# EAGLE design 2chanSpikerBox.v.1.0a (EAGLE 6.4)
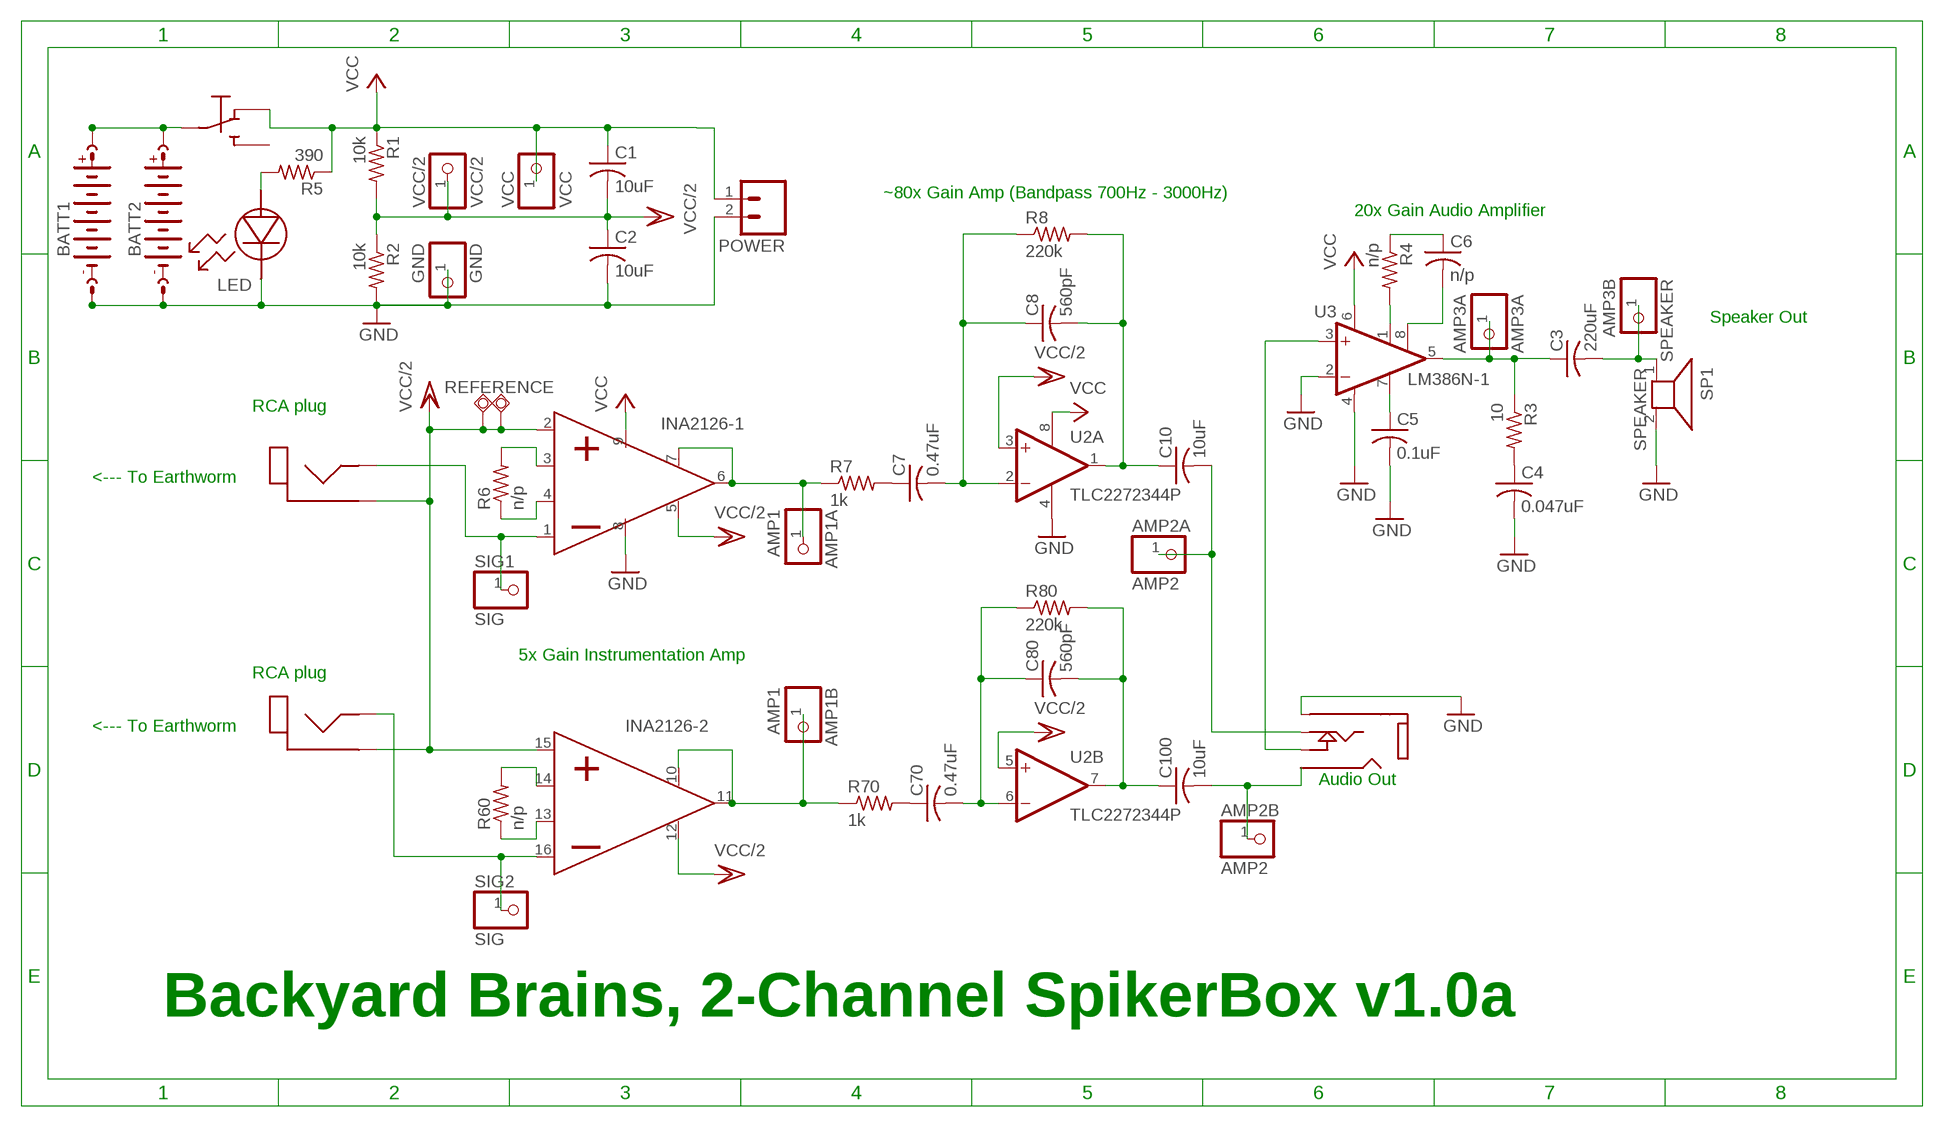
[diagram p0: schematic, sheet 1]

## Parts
AMP1A  AMP1  PINHD-1X1  [1X01]
AMP1B  AMP1  PINHD-1X1  [1X01]
AMP2A  AMP2  PINHD-1X1  [1X01]
AMP2B  AMP2  PINHD-1X1  [1X01]
AMP3A  AMP3A  PINHD-1X1  [1X01]
BATT1  9V-BATT-HOLDERSTANDS  [KEYSTONE-593-594]
BATT2  9V-BATT-HOLDERHEADERS  [1X02]
C1  10uF  C-US050-024X044  [C050-024X044]
C2  10uF  C-US050-024X044  [C050-024X044]
C3  220uF  C-US050-050X075  [C050-050X075]
C4  0.047uF  C-US050-024X044  [C050-024X044]
C5  0.1uF  C-US050-024X044  [C050-024X044]
C6  n/p  C-US050-030X075  [C050-030X075]
C7  0.47uF  C-US050-024X044  [C050-024X044]
C8  560pF  C-US050-024X044  [C050-024X044]
C10  10uF  C-US050-030X075  [C050-030X075]
C70  0.47uF  C-US050-024X044  [C050-024X044]
C80  560pF  C-US050-024X044  [C050-024X044]
C100  10uF  C-US050-030X075  [C050-030X075]
GND  GND  PINHD-1X1  [1X01]
J1  RCA  [RCJ]
J2  RCA  [RCJ]
J4  AUD  AUDIOJACK3.5MM  [AUDIO-JACK]
LED  LEDSSF-LXH104GD  [SSF-LXH104GD]
POWER  M02PTH  [1X02]
R1  10k  R-US_0411/3V  [0411V]
R2  10k  R-US_0411/3V  [0411V]
R3  10  R-US_0309/V  [0309V]
R4  n/p  R-US_0309/V  [0309V]
R5  390  R-US_0309/V  [0309V]
R6  n/p  R-US_0309/V  [0309V]
R7  1k  R-US_0309/V  [0309V]
R8  220k  R-US_0309/V  [0309V]
R60  n/p  R-US_0309/V  [0309V]
R70  1k  R-US_0309/V  [0309V]
R80  220k  R-US_0309/V  [0309V]
REFERENCE  TPSQTP20SQ  [TP20SQ]
REFERENCE1  TPSQTP20SQ  [TP20SQ]
SIG1  SIG  PINHD-1X1  [1X01]
SIG2  SIG  PINHD-1X1  [1X01]
SP1  SPEAKER  [1X02]
SPEAKER  AMP3B  PINHD-1X1  [1X01]
SW1  SWITCH  [SWITCH_THROUGHHOLE]
U1  INA2126  [DIL16]
U2  TLC2272344P  [DIL08]
U3  LM386N-1  [DIL08]
VCC  VCC  PINHD-1X1  [1X01]
VCC/2  VCC/2  PINHD-1X1  [1X01]

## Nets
GND: BATT1.GND$1(-) BATT2.2(-) C2.2 C4.2 C5.2 GND.1 J4.1(SHIELD) LED.CATHODE POWER.2 R2.2 SP1.2 U1.8(PGND) U2.4(A:V-) U3.2(-IN) U3.4(GND)
N$1: AMP2B.1 C100.2 J4.3(INPUTB)
N$2: AMP3A.1 C3.1 R3.1 U3.5(OUT)
N$3: AMP1B.1 R70.1 U1.10(PSENSE) U1.11(POUT)
N$5: C7.1 R7.2
N$6: C4.1 R3.2
N$7: AMP2A.1 C10.2 J4.2(INPUTA)
N$8: C5.1 U3.7(BYPASS)
N$9: C7.2 C8.1 R8.1 U2.2(A:-IN)
N$10: C6.1 R4.1
N$11: R4.2 U3.1(GAIN)
N$12: C6.2 U3.8(GAIN)
N$13: R6.2 U1.3(PG1)
N$14: LED.ANODE R5.2
N$15: J2.SIG SIG2.1 U1.16(P-)
N$16: R6.1 U1.4(PG2)
N$17: AMP1A.1 R7.1 U1.6(POUT) U1.7(PSENSE)
N$18: R60.2 U1.14(PG1)
N$19: C70.1 R70.2
N$20: C70.2 C80.1 R80.1 U2.6(B:-IN)
N$21: J1.SIG SIG1.1 U1.1(P-)
N$22: R60.1 U1.13(PG2)
N$23: C8.2 C10.1 R8.2 U2.1(A:OUT)
N$24: C3.2 SP1.1 SPEAKER.1
N$28: J4.4(SPEAKEROUT) U3.3(+IN)
N$29: C80.2 C100.1 R80.2 U2.7(B:OUT)
V9HOT: BATT1.+9V$1(+) BATT2.1(+) SW1.P2
VCC: C1.1 POWER.1 R1.1 R5.1 SW1.P3 U1.9(PVCC) U2.8(A:V+) U3.6(VS) VCC.1
VCC/2: C1.2 C2.1 J1.GND$1(GND) J2.GND$1(GND) R1.2 R2.1 REFERENCE1.TP REFERENCE.TP U1.2(P+) U1.5(PREF) U1.12(PREF) U1.15(P+) U2.3(A:+IN) U2.5(B:+IN) VCC/2.1
Unconnected: SW1.P1

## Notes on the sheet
- ~80x Gain Amp (Bandpass 700Hz - 3000Hz)
- 20x Gain Audio Amplifier
- Speaker Out
- RCA plug
- INA2126-1
- <--- To Earthworm
- 5x Gain Instrumentation Amp
- RCA plug
- <--- To Earthworm | INA2126-2
- Audio Out
- Backyard Brains, 2-Channel SpikerBox v1.0a

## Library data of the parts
AMP1A AMP1B AMP2A AMP2B AMP3A GND SIG1 SIG2 SPEAKER VCC VCC/2 = pinhead:PINHD-1X1: PIN HEADER
BATT1 = byb:9V-BATT-HOLDER; DIGIKEY: 593K-ND, 594K-ND; MANUFACTURER: KEYSTONE ELECTRONICS; PARTNO: 593,594
BATT2 = byb:9V-BATT-HOLDER; DIGIKEY: N145-ND; MANUFACTURER: ENERGIZER BATTERY COMPANY; PARTNO: EN22
C1 C2 = resistor:C-US: CAPACITOR, American symbol; DIGIKEY: P986-ND; MANUFACTURER: Panasonic - ECG; PARTNO: ECE-A1HKSR22
C3 = resistor:C-US: CAPACITOR, American symbol; DIGIKEY: 565-1674-ND; MANUFACTURER: UNITED CHEMI-CON; PARTNO: EKZE250ELL221MHB5D
C4 = resistor:C-US: CAPACITOR, American symbol; DIGIKEY: BC1099CT-ND; MANUFACTURER: VISHAY/BC COMPONENTS; PARTNO: K473K15X7RF5TH5
C5 = resistor:C-US: CAPACITOR, American symbol; DIGIKEY: BC1148CT-ND; MANUFACTURER: Vishay/BC Components; PARTNO: K104Z15Y5VE5TL2
C6 C10 C100 = resistor:C-US: CAPACITOR, American symbol; DIGIKEY: P966-ND; MANUFACTURER: Panasonic - ECG; PARTNO: ECE-A1CKS100
C7 C70 = resistor:C-US: CAPACITOR, American symbol; DIGIKEY: BC1150CT-ND; MANUFACTURER: Vishay/BC Components; PARTNO: K474Z20Y5VE5TL2
C8 C80 = resistor:C-US: CAPACITOR, American symbol; DIGIKEY: BC1022CT-ND; MANUFACTURER: Vishay/BC Components; PARTNO: K561J15C0GF5TL2
J1 J2 = byb:RCA: RCA Edge Connector; DIGIKEY: CP-1403-ND; MANUFACTURER: CUI Inc; PARTNO: RCJ-014
J4 = byb:AUDIOJACK: 1/8" Audio Jack; DIGIKEY: CP1-3524NG-ND; MANUFACTURER: CUI Inc; PARTNO: SJ1-3524NG
LED = byb:LED: SIDE LED (Green); DIGIKEY: 67-1037-ND; MANUFACTURER: LUMEX OPTO/COMPONENTS INC; PARTNO: SSF-LXH104GD
POWER = SparkFun:M02: Header 2
R1 R2 = resistor:R-US_: RESISTOR, American symbol; DIGIKEY: P10KBACT-ND; MANUFACTURER: Panasonic - ECG; PARTNO: ERD-S2TJ103V
R3 = resistor:R-US_: RESISTOR, American symbol; DIGIKEY: P10BACT-ND; MANUFACTURER: Panasonic - ECG; PARTNO: ERD-S2TJ100V
R4 = resistor:R-US_: RESISTOR, American symbol; DIGIKEY: CD14ZT0R00CT-ND; MANUFACTURER: Stackpole Electronics; PARTNO: CD14ZT0R00
R5 = resistor:R-US_: RESISTOR, American symbol; DIGIKEY: CF14JT390RCT-ND; MANUFACTURER: Stackpole Electronics; PARTNO: CF14JT390R
R6 R60 = resistor:R-US_: RESISTOR, American symbol; DIGIKEY: P68KBACT-ND; MANUFACTURER: Panasonic - ECG; PARTNO: ERD-S2TJ683V
R7 R70 = resistor:R-US_: RESISTOR, American symbol; DIGIKEY: P1.0KBACT-ND; MANUFACTURER: Panasonic - ECG; PARTNO: ERD-S2TJ102V
R8 R80 = resistor:R-US_: RESISTOR, American symbol; DIGIKEY: P220KCACT-ND; MANUFACTURER: Panasonic - ECG; PARTNO: ERO-S2PHF2203
REFERENCE REFERENCE1 = testpad:TPSQ: Test pad
SP1 = byb:SPEAKER: SPEAKER; DIGIKEY: 102-1554-ND; MANUFACTURER: CUI Inc; PARTNO: CLS0271M-L152
SW1 = byb:SWITCH: Toggle Switch
U1 = byb:INA2126
U2 = byb:TLC2272: Dual Operational Amplifier Low Power, Single-Supply, Rail-To-Rail Operational Amplifier Source: http://focus.ti.com/lit/ds/symlink/opa2345.pdf http://focus.ti.com .. opa241.pdf http://focus.ti.com/lit/ds/symlink/opa2134.pdf; DIGIKEY: 296-1812-5-ND; MANUFACTURER: TEXAS INSTRUMENTS; PARTNO: TLC2272CP
U3 = byb:LM386?-*: Low Voltage Audio Power Amplifier Source: http://cache.national.com/ds/LM/LM386.pdf; DIGIKEY: LM386N-3-ND; MANUFACTURER: NATIONAL SEMICONDUCTOR; PARTNO: LM386N-3/NOPB

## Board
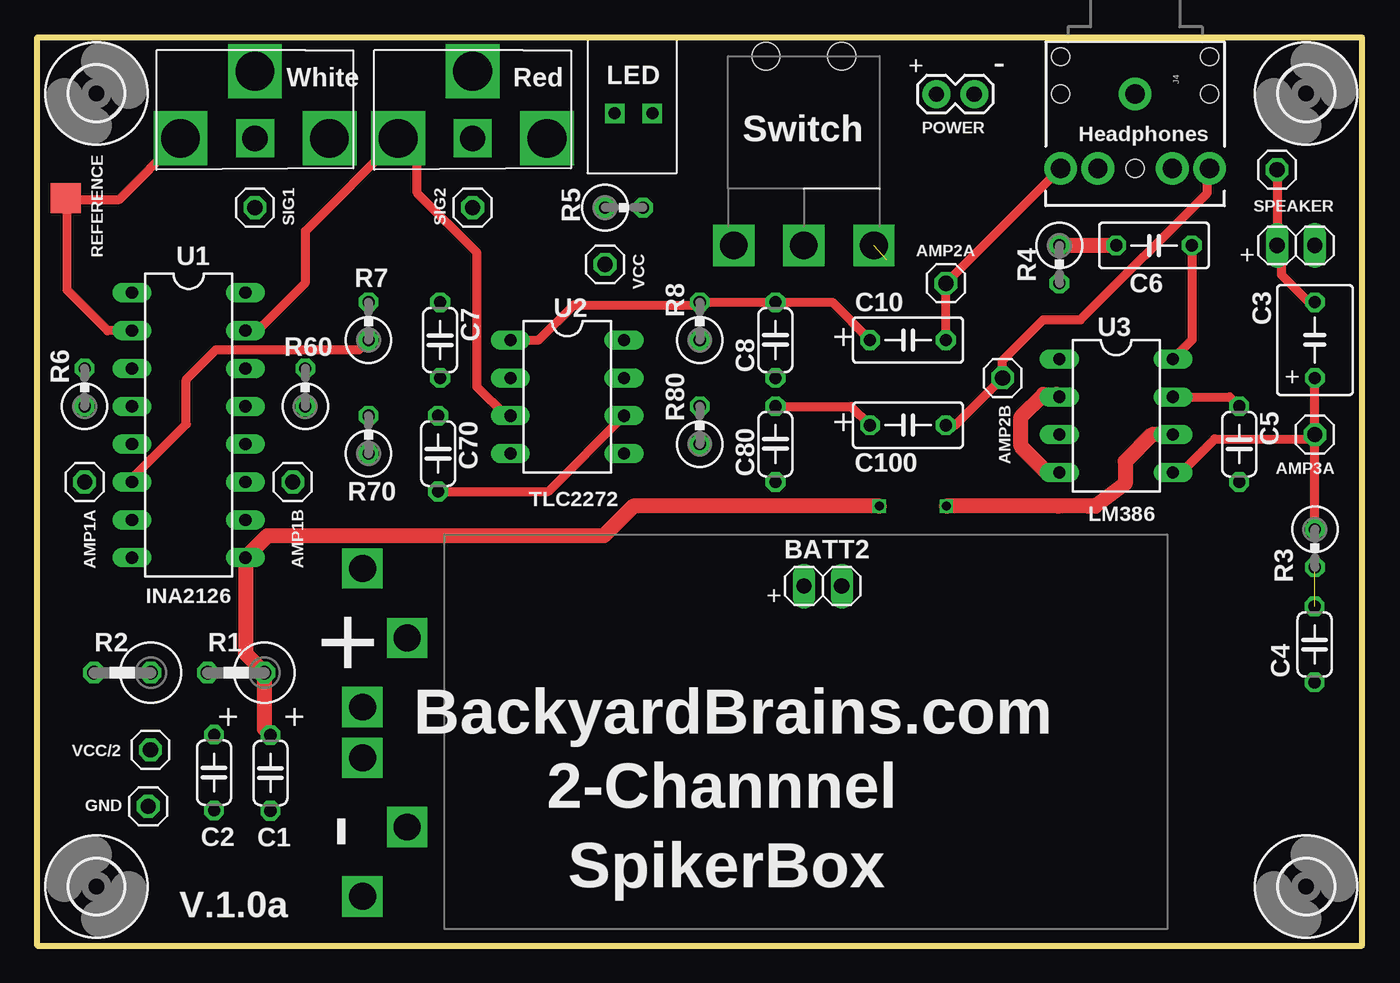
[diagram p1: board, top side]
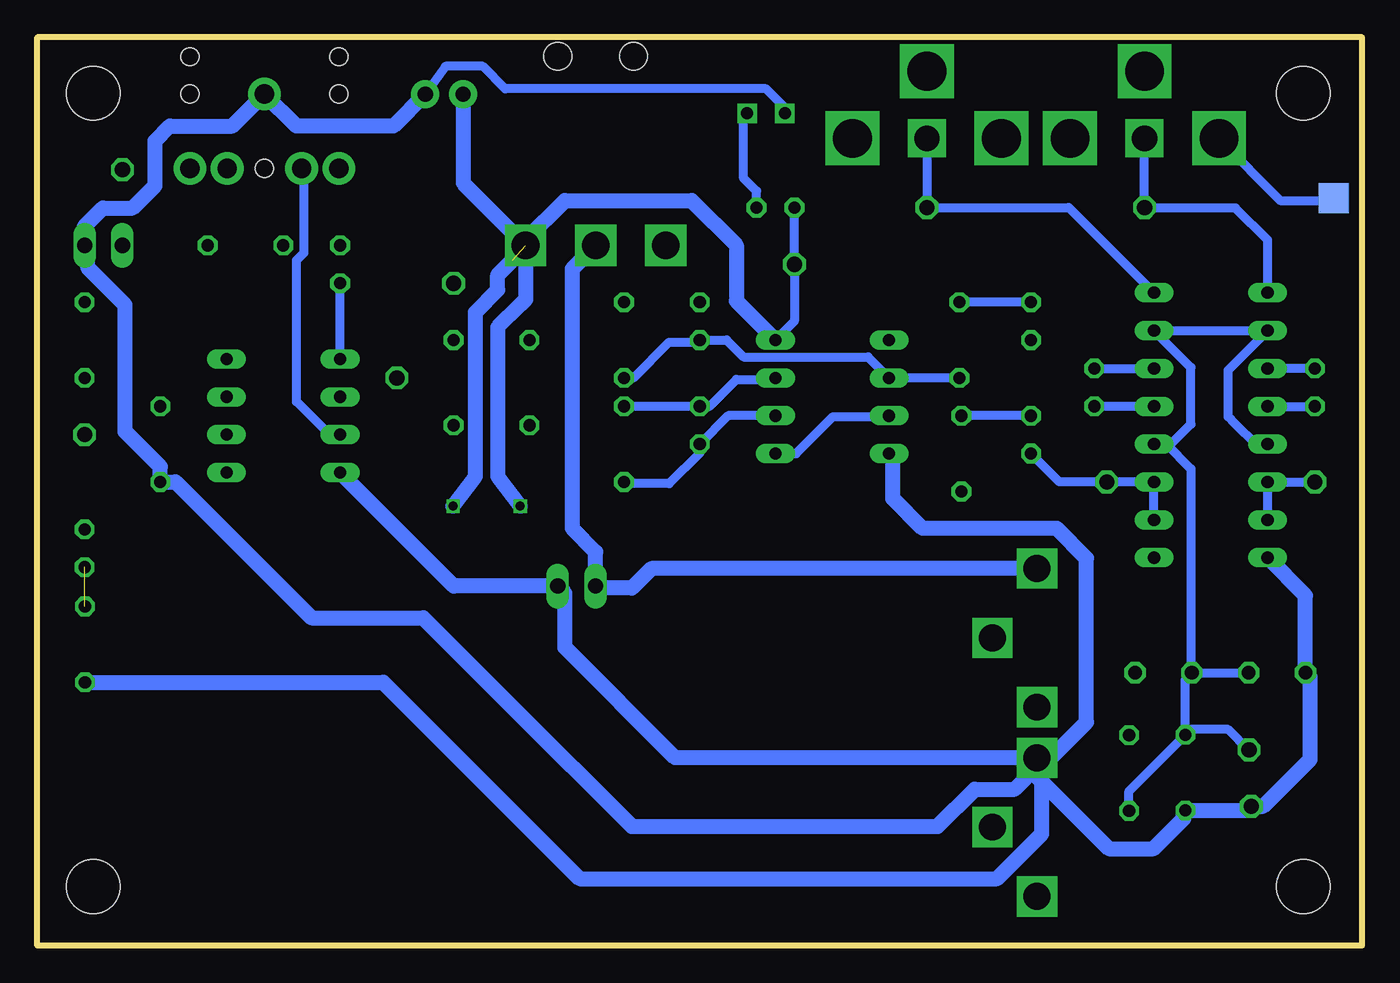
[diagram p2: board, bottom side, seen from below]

Size 88.9 x 60.96 mm. Coordinates in mm from the lower left corner, seen from the top.
Outline: 0,0 0,60.96 88.9,60.96 88.9,0 0,0
Copper layers (1*16): Top 0.035mm / dielectric 1.5mm / Bottom 0.035mm
Design rules "default": minimum track width 6mil, minimum drill 12mil, track to track 6mil, track to pad 6mil, pad to pad 6mil, via to via 6mil, smd to smd 0mil, copper to edge 10mil, drill to drill 10mil, minimum pad ring 10mil, minimum via ring 6mil, stop-mask expansion 2mil, vias tented up to drill 100mil, thermal gap 10mil

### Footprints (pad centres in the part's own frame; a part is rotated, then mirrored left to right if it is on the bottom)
1X01 = drill 1.016 octagon: 1 0,0
KEYSTONE-593-594 = drill 1.8 square: +9V$1 -10.7,1.5; +9V$2 -6.05,4.5; +9V$3 -1.4,1.5; GND$1 2,1.5; GND$2 6.65,4.5; GND$3 11.3,1.5
1X02 = drill 1.016 long: 1 -1.27,0; 2 1.27,0
C050-024X044 = drill 0.813 octagon: 1 -2.54,0; 2 2.54,0
C050-050X075 = drill 0.813 octagon: 1 -2.54,0; 2 2.54,0
C050-030X075 = drill 0.813 octagon: 1 -2.54,0; 2 2.54,0
3,6 = hole 3.6: 0,0
RCJ = drill 2.6 square: GND$1 -5,-4.5; GND$2 0,0; GND$3 5,-4.5 | drill 1.7 square: SIG 0,-4.5
AUDIO-JACK = drill 1.3 pad 2.184: 1 0,0; 2 5,-5; 3 5,5; 4 5,-2.5; 5 5,2.5 | hole 1.2: 0,5; -2.5,5; -2.5,-5; 0,-5; 5,0
SSF-LXH104GD = drill 0.8 square: ANODE 5.1,1.27; CATHODE 5.1,-1.27
1X02' = drill 1.016 pad 1.88: 1 0,0; 2 2.54,0
0411V = drill 0.914 octagon: 1 -2.54,0; 2 1.27,0
0309V = drill 0.813 octagon: 1 -1.27,0; 2 1.27,0
TP20SQ = smd 2 x 2: TP 0,0
SWITCH_THROUGHHOLE = drill 1.85 square: P1 0,-4.7; P2 0,0; P3 0,4.7 | hole 1.85: -12.7,2.54; -12.7,-2.54
DIL16 = drill 0.813 long: 1 -8.89,-3.81; 2 -6.35,-3.81; 3 -3.81,-3.81; 4 -1.27,-3.81; 5 1.27,-3.81; 6 3.81,-3.81; 7 6.35,-3.81; 8 8.89,-3.81; 9 8.89,3.81; 10 6.35,3.81; 11 3.81,3.81; 12 1.27,3.81; 13 -1.27,3.81; 14 -3.81,3.81; 15 -6.35,3.81; 16 -8.89,3.81
DIL08 = drill 0.813 pad 1.27 long: 1 -3.81,-3.81; 2 -1.27,-3.81; 3 1.27,-3.81; 4 3.81,-3.81; 5 3.81,3.81; 6 1.27,3.81; 7 -1.27,3.81; 8 -3.81,3.81

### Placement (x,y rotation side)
AMP1A  3.17,31.11 270 top
AMP1B  17.14,31.11 0 top
AMP2A  60.96,44.45 90 top
AMP2B  64.77,38.1 270 top
AMP3A  85.72,34.29 180 top
BATT1  20.32,14.61 270 top
BATT2  52.7,24.13 0 top
C1  15.65,11.59 270 top
C2  11.86,11.61 270 top
C3  85.72,40.64 90 top
C4  85.7,20.22 270 top
C5  80.64,33.66 270 top
C6  74.93,46.99 0 top
C7  27.03,40.64 270 top
C8  49.53,40.64 90 top
C10  58.42,40.64 0 top
C70  26.9,33.02 270 top
C80  49.53,33.66 90 top
C100  58.42,34.92 0 top
GND  7.44,9.35 180 top
H1  MOUNT-HOLE3.6  [3,6]  85.14,57.2 0 top
H2  MOUNT-HOLE3.6  [3,6]  3.96,57.2 0 top
H3  MOUNT-HOLE3.6  [3,6]  85.14,3.96 0 top
H4  MOUNT-HOLE3.6  [3,6]  3.96,3.96 90 top
J1  14.61,58.67 0 top
J2  29.21,58.67 0 top
J4  73.66,57.15 270 top
LED  40.01,60.96 270 top
POWER  [1X02']  60.33,57.15 0 top
R1  12.7,18.32 180 top
R2  5.08,18.32 180 top
R3  85.72,26.67 270 top
R4  68.58,45.72 270 top
R5  39.37,49.53 0 top
R6  3.17,37.47 90 top
R7  22.23,41.91 90 top
R8  44.45,41.91 90 top
R60  17.98,37.47 90 top
R70  22.23,34.29 90 top
R80  44.45,34.92 90 top
REFERENCE  1.91,50.16 0 top
REFERENCE1  1.91,50.16 0 bottom
SIG1  14.61,49.53 180 top
SIG2  29.21,49.53 180 top
SP1  84.45,46.99 0 top
SPEAKER  83.19,52.07 0 top
SW1  51.44,46.99 270 top
U1  10.16,34.92 270 top
U2  35.56,36.83 270 top
U3  72.39,35.56 270 top
VCC  38.1,45.72 270 top
VCC/2  7.59,13.14 270 top

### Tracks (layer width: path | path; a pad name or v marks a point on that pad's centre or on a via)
GND
  Top 1: U3.4 67.75,31.75 66,33.5 66,35.5 67.5,37 68.41,37 U3.2
  Bottom 0.61: LED.CATHODE 38.73,56.23 40,57.5 57.5,57.5 59,59 61.52,59 POWER.2
  Bottom 1: BATT1.GND$1 21.82,12 | 21.82,12 21.82,11.32 17,6.5 14,6.5 13.5,7 12,8.5 12,8.94 C2.2 7.72,9.07 GND.1 6.65,9.35 3.5,12.5 3.5,18.01 R2.2 3.81,23.5 U1.8 | BATT1.GND$1 46.1,12.61 53.5,20 53.5,23.66 BATT2.2 60.96,24.13 U3.4 | BATT1.GND$1 20.89,12.61 18.5,15 18.5,26 20.5,28 29.5,28 31.5,30 31.5,32.77 U2.4 | POWER.2 62.87,57.13 65,55 71.51,55 J4.1 75.81,55 80,55 81,54 81,53.5 81,51 81.5,50.5 82.5,49.5 84.5,49.5 85.72,48.27 SP1.2 85.5,46.77 85.5,45.5 83,43 83,34.5 80.64,32.15 C5.2 79.61,31.11 70.5,22 63,22 57,16 49,8 28.5,8 26,10.5 23.32,10.5 21.82,12 | C4.2 65.68,17.68 52.5,4.5 24.5,4.5 23.5,5.5 21.5,7.5 21.5,11.68 21.82,12
N$1
  Top 0.61: C100.2 61.59,34.92 AMP2B.1 64.77,39.27 67.5,42 70,42 78.5,50.5 78.5,51.99 J4.3
N$2
  Top 0.61: U3.5 76.75,31.75 79,34 85.44,34 AMP3A.1 | AMP3A.1 C3.1 | R3.1 AMP3A.1
N$3
  Bottom 0.61: U1.10 U1.11 AMP1B.1 20.32,31.11 R70.1
N$5
  Bottom 0.61: R7.2 C7.1
N$6  (1 unrouted)
N$7
  Top 0.61: C10.2 AMP2A.1 J4.2
N$8
  Top 0.61: U3.7 80.01,36.83 C5.1
N$9
  Bottom 0.61: C7.2 U2.2 33.15,39.5 41.5,39.5 42.64,40.64 R8.1 44.59,40.5 46.5,40.5 48.9,38.1 C8.1
N$10
  Top 1: C6.1 R4.1
N$11
  Bottom 0.61: U3.1 R4.2
N$12
  Top 0.61: C6.2 77.47,40.64 U3.8
N$13
  Bottom 0.61: R6.2 U1.3
N$14
  Bottom 0.61: R5.2 40.64,50.64 41.5,51.5 41.5,55.63 LED.ANODE
N$15
  Bottom 0.61: J2.SIG SIG2.1 19.68,49.53 U1.16
N$16
  Bottom 0.61: U1.4 R6.1
N$17
  Top 0.61: U1.6 6.35,31.35 10,35 10,38 12,40 21.59,40 R7.1
  Bottom 0.61: AMP1A.1 U1.6 U1.7
N$18
  Bottom 0.61: R60.2 U1.14
N$19
  Bottom 0.61: R70.2 C70.1
N$20
  Top 0.61: C70.2 34.29,30.48 U2.6
  Bottom 0.61: U2.6 42.55,35.56 R80.1 44.45,33.05 46.5,31 49.41,31 C80.1
N$21
  Bottom 0.61: U1.1 6.35,47.35 8.5,49.5 14.57,49.5 SIG1.1 J1.SIG
N$22
  Bottom 0.61: U1.13 R60.1
N$23
  Top 0.61: U2.1 33.64,40.64 36,43 44.27,43 R8.2 C8.2 53.34,43.18 C10.1
N$24
  Top 0.61: SPEAKER.1 SP1.1 83.5,46.67 83.5,45 85.32,43.18 C3.2
N$28
  Bottom 0.61: U3.3 69.29,34.29 71.5,36.5 71.5,46 71,46.5 71,51.99 J4.4
N$29
  Top 0.61: C80.2 54.61,36.2 C100.1
  Bottom 0.61: U2.7 39.47,38 42,38 43.8,36.2 R80.2 C80.2
V9HOT
  Bottom 1: BATT1.+9V$1 47.7,25.3 49,24 51.3,24 BATT2.1 51.44,26.43 53,28 53,45.42 SW1.P2
VCC  (via drill 0.6)  (1 unrouted)
  Top 1: v56.5,29.5 40,29.5 38,27.5 15.44,27.5 U1.9 13.97,19.59 R1.1 15.24,14.54 C1.1 | U3.6 74.79,34.29 73,32.5 73,31 71,29.5 70.5,29.5 68.5,29.5 v61,29.5
  Bottom 0.61: U2.8 38.1,41.91 VCC.1 R5.1
  Bottom 1: POWER.1 60.33,51.18 SW1.P3 | SW1.P3 56.13,47.37 53.5,50 45,50 42,47 42,43.27 U2.8 | SW1.P3 56.13,43.37 56.5,43 58,41.5 58,31.5 v56.5,29.5 | v61,29.5 59.5,31.5 59.5,32.5 59.5,42.5 58,44 58,45 57,46
VCC/2
  Top 0.61: U1.2 4.72,41.27 2,44 2,50.07 | 2,50.07 REFERENCE1.TP | 2,50.07 5.5,50.07 J1.GND$1 | U2.3 31.44,35.56 29.5,37.5 29.5,46.5 25.5,50.5 25.5,52.88 J2.GND$1 18,47.96 18,44.5 14.78,41.27 U1.15
  Bottom 0.61: J1.GND$1 9.61,54.1 5.5,50 2.07,50 REFERENCE1.TP | U1.5 7.16,33.66 8.5,35 9,35.5 9,38.5 9,38.62 U1.2 U1.15 11.5,38.8 11.5,35 12.85,33.66 U1.12 13.15,33.66 11.5,32 11.5,18.39 R1.2 | R1.2 R2.1 | VCC/2.1 7.64,13.14 9,14.5 11.52,14.5 C2.1 | C1.2 15.65,10.37 C2.1 | C2.1 11.86,17.89 R1.2 | U2.5 37.98,33.02 35.5,35.5 31.81,35.5 U2.3

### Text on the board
tPlace: + | BackyardBrains.com | 2-Channnel | SpikerBox
tNames: White | Red | LED | - | Switch | Headphones | + | + | + | TLC2272 | LM386 | INA2126 | + | + | V.1.0a
201bmp: http://backyardbrains.com | Backyard Brains | 2 Channel | SpikerBox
